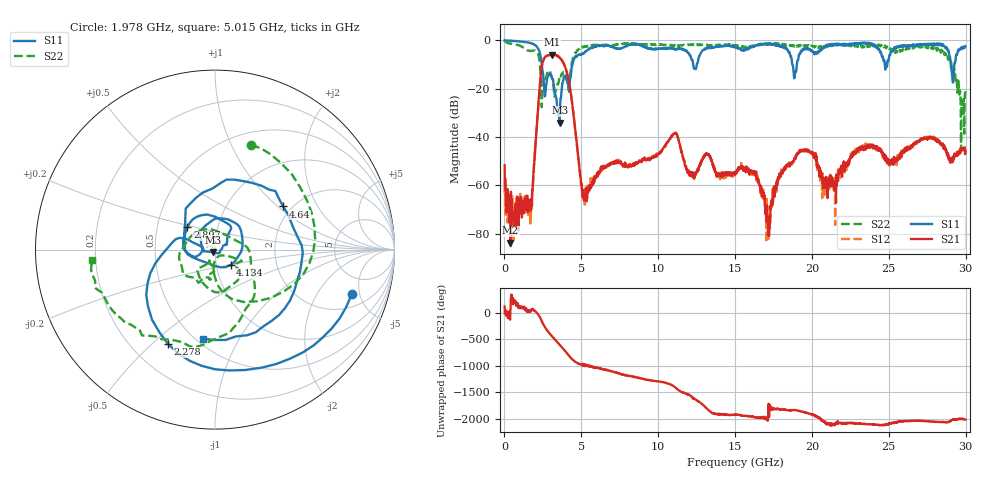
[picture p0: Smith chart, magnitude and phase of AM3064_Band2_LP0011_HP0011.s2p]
# Hz S DB R 50.0
!freq dBS11 angS11 dBS21 angS21 dBS12 angS12 dBS22 angS22
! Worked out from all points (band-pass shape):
!   1600 points, 10 MHz to 29.98 GHz, reference 50 ohm
!   highest |S21| = -5.88 dB at 3.084 GHz (marker M1); lowest = -83.8 dB at 384.9 MHz (marker M2)
!   |S21| within 3 dB of the highest: 2.5 GHz to 3.798 GHz (1.298 GHz wide, 41.2 % of centre)
!   lowest |S11| = -34.1 dB at 3.59 GHz (marker M3), VSWR 1.04, Z = 48.9 - j1.57 ohm
!   |S11| at or under -10 dB: 2.421 GHz to 4.424 GHz (2.003 GHz wide, 58.5 % of centre); 12.28 GHz to 12.52 GHz (240.8 MHz wide, 1.94 % of centre); 18.73 GHz to 19.02 GHz (293.7 MHz wide, 1.56 % of centre)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
!   |S22| runs from -45.4 to -0.2 dB; largest |S21 - S12| = 0.013
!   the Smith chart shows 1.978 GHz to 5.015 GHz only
!   S11 on the Smith chart (normalised r, x): 1.978 GHz: 3.03, -4.20; 2.278 GHz: 0.35, -0.56; 2.897 GHz: 0.71, +0.19; 4.134 GHz: 1.17, -0.20; 4.64 GHz: 1.80, +1.09; 5.015 GHz: 0.54, -0.72
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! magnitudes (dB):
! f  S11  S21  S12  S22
! 10 MHz  0.0  -51.7  -60.3  -0.2
! 384.9 MHz  -0.2  -83.8  -69.0  -1.4
! 1.678 GHz  -1.1  -68.2  -76.7  -4.4
! 1.978 GHz  -1.9  -47.1  -46.5  -4.2
! 2.278 GHz  -4.6  -20.3  -20.3  -8.6
! 2.897 GHz  -14.1  -6.2  -6.1  -12.4
! 3.084 GHz  -15.5  -5.9  -5.8  -15.6
! 3.59 GHz  -34.1  -7.1  -7.2  -15.4
! 4.134 GHz  -18.3  -15.3  -15.3  -19.0
! 4.64 GHz  -6.9  -38.8  -38.7  -5.2
! 5.015 GHz  -6.0  -59.4  -59.5  -3.3
! 10 GHz  -3.5  -46.9  -47.0  -1.8
! 15 GHz  -2.6  -55.4  -55.1  -1.9
! 16.3 GHz  -2.2  -55.0  -55.5  -2.1
! 17.18 GHz  -1.8  -78.6  -77.6  -1.5
! 18.06 GHz  -2.2  -55.3  -54.3  -1.8
! 19.99 GHz  -4.2  -46.4  -46.9  -2.2
! 20.82 GHz  -2.5  -60.3  -60.7  -2.3
! 25 GHz  -8.0  -49.4  -50.6  -2.8
! 28.56 GHz  -2.2  -43.7  -43.8  -4.7
! 29.18 GHz  -17.5  -49.1  -48.7  -10.3
! 29.98 GHz  -2.5  -46.0  -46.0  -21.6
